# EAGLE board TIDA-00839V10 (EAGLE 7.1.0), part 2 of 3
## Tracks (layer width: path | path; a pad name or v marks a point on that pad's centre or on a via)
+5..12V
  Top 0.406: U7.3 31.36,165.84 29.82,165.84 C70.1 | U7.1 30.01,167.79 29.74,167.52 29.74,165.92 C70.1 | C70.1 29.67,165.8 D51.1 28.23,165.76 D50.1 28.26,163.91 C69.1
ACT
  Top 0.254: MSP430F67791A.29 127.51,107.38 129.01,108.88 129.01,115.62 127.26,117.38 123.01,117.38 121.51,118.88 121.51,140.62 111.01,151.12 111.01,162.62 102.76,170.88 78.43,170.88 LED_ACT.K
  Top 0.61: U8.2 110.45,181.33 108.48,183.29 96.98,183.29 93.32,179.64 74.61,179.64 JP12.1
  Bottom 0.254: 76.36,168.72 LED_ACT.K 76.32,168.77 76.32,172.5 73.09,175.73 70.96,175.73 JP12.1
AUXVCC1  (via drill 0.2, 0.4, 0.5)
  Top 0.254: v121.26,89.03 120.01,90.28 MSP430F67791A.124 120.01,98.84 108.91,109.94 v108.89,109.94 | v128.51,87.62 C26.1 | C27.1 130.66,85.22 v131.51,84.38
  Top 0.406: C26.1 128.51,84.88 128.86,85.22 C27.1
  Top 0.61: R4.2 87.17,117.8 C58.1 89.85,117.8 v89.86,117.81
  Top 0.813: R62.2 139.8,81.03 SV1.6
  Bottom 0.254: v128.51,87.62 122.66,87.62 v121.26,89.03 | v89.86,117.81 106.96,117.81 108.86,115.91 108.86,109.97 v108.89,109.94
  Bottom 0.61: v131.51,84.38 131.47,84.34 137.36,84.34 SV1.6
AUXVCC2  (via drill 0.2)
  Top 0.254: MSP430F67791A.123 119.51,89.88 v120.26,89.12 | C24.1 v125.51,86.62
  Top 0.406: C24.1 125.51,85.38 125.66,85.22 C25.1
  Bottom 0.254: v125.51,86.62 122.76,86.62 v120.26,89.12
  Bottom 0.61: v125.51,86.62 137.61,86.62 SV1.4
AUXVCC3  (via drill 0.3, 0.36, 0.4)
  Top 0.254: C43.1 128.13,97 | MSP430F67791A.3 124.76,94.38 127.41,97.03 C43.1 | C43.1 128.01,96.88 128.16,97.03 C44.1 130.16,97.03 v131.51,98.38 | v142.76,93.12 142.76,89.62 145.31,87.07 SV1.2 | R49.1 131.36,136.31 132.05,135.62 133.45,135.62 v138.66,130.41
  Top 0.406: R52.1 132.02,157.88 132.81,157.08 132.81,138.83 R49.1
  Bottom 0.254: v131.51,98.38 138.81,98.38 142.71,94.47 142.71,93.17 v142.76,93.12 142.81,93.07 144.5,93.07 145.31,93.89 145.31,128.46 143.36,130.41 v138.66,130.41
AVCC  (via drill 0.6)
  Top 0.254: 117.76,85.62 117.86,85.53 C29.1 | 118.01,86.88 117.96,86.83 C31.1 | MSP430F67791A.121 118.51,90.2 118.01,89.7 118.01,86.83 C31.1 | C31.1 117.81,86.83 117.76,86.88 117.91,87.03
  Top 0.406: C29.1 118.01,85.62 117.91,85.72 | 122.51,68.88 122.5,68.88
  Top 0.61: 122.5,68.88 116.51,74.88 116.51,78.88 117.86,80.22 | 122.51,68.88 139.26,68.88 143.26,64.88 v143.26,43.38 | 117.91,85.72 C31.1 | 117.86,80.22 117.86,85.53 | R36.2 119.2,78.89 117.86,80.22 | D36.C 127.83,43.45 v127.76,43.38 127.68,43.45 D34.C | 112.93,43.33 D32.C | v112.88,43.38 110.71,43.38 D30.C | 98.08,43.45 D28.C | 97.93,43.45 D42.C | v83.01,43.38 85.43,43.38 D40.C
  Top 0.813: D30.C 110.51,43.38 | v143.26,43.38 140.18,43.38 D38.C | 98.08,43.45 v98.01,43.38 97.93,43.45 | v112.88,43.38 112.93,43.33
  Bottom 0.61: v143.26,43.38 v127.76,43.38 v112.88,43.38 v98.01,43.38 v83.01,43.38
BTN1  (via drill 0.2, 0.4)
  Top 0.254: v121.51,98.38 MSP430F67791A.11 | R53.2 139.62,158.13 | R53.2 139.36,162.58 DBTN1.2 | R53.2 139.36,155.03 v139.51,154.88
  Bottom 0.254: v121.51,98.38 121.51,102.38 123.51,104.38 134.01,104.38 136.51,106.88 136.51,131.88 138.01,133.38 138.01,153.38 v139.51,154.88
BTN2  (via drill 0.2, 0.36)
  Top 0.254: MSP430F67791A.10 122.01,97.88 v121.51,97.38 | DBTN2.2 139.36,141.88 R50.2 139.36,136.22 v137.01,133.88
  Bottom 0.254: v121.51,97.38 121.01,97.38 120.51,97.88 120.51,102.62 123.26,105.38 133.51,105.38 135.51,107.38 135.51,132.38 v137.01,133.88
BTN3  (via drill 0.2, 0.36)
  Top 0.254: MSP430F67791A.4 123.01,94.88 v121.51,93.38 | ABTN3.2 129.66,141.78 R49.2 129.66,136.22 v132.01,133.88
  Bottom 0.254: v121.51,93.38 120.76,93.38 119.51,94.62 119.51,96.38 118.51,97.38 118.51,103.12 122.76,107.38 132.51,107.38 133.51,108.38 133.51,132.38 v132.01,133.88
BTN4  (via drill 0.2, 0.4)
  Top 0.254: MSP430F67791A.5 122.51,95.38 v121.51,94.38 | R52.2 130.01,158.23 | R52.2 129.66,162.49 ABTN4.2 | R52.2 129.66,156.22 v131.01,154.88
  Bottom 0.254: v121.51,94.38 121.01,94.38 120.51,94.88 120.51,96.62 119.51,97.62 119.51,102.88 123.01,106.38 133.01,106.38 134.51,107.88 134.51,132.88 133.01,134.38 133.01,152.88 v131.01,154.88
COM0  (via drill 0.2)
  Top 0.254: MSP430F67791A.22 121.01,103.88 v113.51,111.38 | LCD1.COM0 94.38,162.5 v109.26,147.62
  Bottom 0.254: v113.51,111.38 113.51,143.38 v109.26,147.62
COM1  (via drill 0.2)
  Top 0.254: MSP430F67791A.23 121.51,104.38 v114.51,111.38 | v109.26,149.12 109.26,149.15 96.62,161.78 96.62,162.46 LCD1.COM1
  Bottom 0.254: v114.51,111.38 114.51,143.88 v109.26,149.12
COM2  (via drill 0.2)
  Top 0.254: MSP430F67791A.24 122.01,104.88 v115.51,111.38 | LCD1.COM2 99.2,160.68 v109.26,150.62
  Bottom 0.254: v115.51,111.38 115.51,144.38 v109.26,150.62
COM3  (via drill 0.2)
  Top 0.254: MSP430F67791A.25 122.51,105.38 v116.51,111.38 | v109.26,152.12 109.26,152.19 101.7,159.75 101.7,162.46 LCD1.COM3
  Bottom 0.254: v116.51,111.38 116.51,144.88 v109.26,152.12
CUR1+
  Top 0.406: 104.04,53.12 TVS2.C 104.03,54.12 103.95,54.2 | D11.C 104.04,50.95
  Top 0.61: 103.95,54.2 103.96,54.2 R/L9.2
  Top 0.679: D3.A D11.C | 104.04,50.95 104.04,53.12
  Top 0.813: D3.A 103.96,33.36 I1+.TP
CUR1-
  Top 0.406: 107.14,53.12 TVS2.A 107.15,54.12 107.07,54.2 | D12.C 107.14,50.95
  Top 0.61: 107.07,54.2 107.06,54.2 R/L10.2
  Top 0.679: D4.A D12.C | 107.14,50.95 107.14,53.12
  Top 0.813: D4.A 107.06,33.41 I1-.TP
CUR2+
  Top 0.406: TVS3.C 118.73,53.99 | 118.73,53.99 118.86,54.12 | 118.73,53.99 118.86,54.12
  Top 0.61: 118.86,54.12 118.83,54.12 R/L11.2 | D13.C 118.83,53.12 TVS3.C
  Top 0.679: D5.A D13.C
  Top 0.813: D5.A 118.83,33.41 I2+.TP
CUR2-
  Top 0.406: TVS3.A 121.98,54.12 | TVS3.A 121.97,53.12 121.93,53.09 | TVS3.A 121.94,54.12
  Top 0.61: 121.98,54.12 121.93,54.12 R/L12.2
  Top 0.679: D6.A D14.C 121.93,53.09
  Top 0.813: D6.A 121.93,33.36 I2-.TP
CUR3+
  Top 0.406: 133.7,54.12 TVS4.C 133.71,53.12
  Top 0.61: 133.7,54.12 133.71,54.12 R/L13.2
  Top 0.679: 133.71,53.12 D15.C D7.A
  Top 0.813: D7.A 133.71,33.47 I3+.TP
CUR3-
  Top 0.406: 136.82,54.12 TVS4.A 136.81,53.12
  Top 0.61: 136.82,54.12 136.81,54.12 R/L14.2
  Top 0.679: 136.81,53.12 D16.C D8.A
  Top 0.813: D8.A 136.81,33.3 I3-.TP
CURN+
  Top 0.406: 88.94,53.12 TVS1.C 88.86,54.02 | 88.86,54.02 88.95,54.12 | 88.96,53.92 88.86,54.02
  Top 0.61: 88.95,54.12 88.96,54.12 R/L7.2
  Top 0.679: D1.A D9.C 88.96,53.92
  Top 0.813: D1.A 88.96,33.31 IN+.TP
CURN-
  Top 0.406: 92.16,53.24 92.04,53.12 | 92.16,53.24 TVS1.A 92.07,54.12 | 92.06,53.14 92.16,53.24
  Top 0.61: 92.07,54.12 92.06,54.12 R/L8.2
  Top 0.679: D2.A D10.C 92.06,53.14
  Top 0.813: D2.A 92.06,33.45 IN-.TP
DRESET  (via drill 0.36)
  Top 0.254: v49.01,120.88 49.51,120.38 89.51,120.38 91.01,118.88 91.01,102.88 v91.13,102.75 | MSP430F67791A.102 106.51,93.38 v104.63,91.5
  Bottom 0.254: JP5.2 27.99,127.81 42.08,127.81 v49.01,120.88 | v91.13,102.75 91.13,96.75 96.38,91.5 v104.63,91.5
DRV1GND
  Top 0.254: MSP430F67791A.20 148.39,102.88 152.73,98.53
  Top 0.61: U1GND.1 36.38,2.54 37.11,1.81 124.41,1.81 152.73,30.13 152.73,98.53
DRV2GND
  Top 0.254: MSP430F67791A.18 146.49,101.88 150.75,97.62
  Top 0.61: U2GND.1 63.15,5.24 64.89,3.49 123.11,3.49 150.75,31.12 150.75,97.62
DRV3GND
  Top 0.254: MSP430F67791A.12 126.3,98.88 127.33,99.91 143.23,99.91 147.62,95.51
  Top 0.61: U3GND.1 100.68,7.05 100.96,6.77 121.46,6.77 147.57,32.88 147.57,95.46 147.62,95.51
DRV4GND
  Top 0.254: MSP430F67791A.95 95.09,96.88 90.63,92.41 90.63,75.78 90.09,75.24 67.21,75.24 66.57,75.88 66.57,76.97 65.7,77.84 U4GND.1
DRV5GND
  Top 0.254: MSP430F67791A.93 94.16,97.88 89.46,93.18 89.46,78.32 88.39,77.25 U5GND.1
DRV6GND
  Top 0.254: U6GND.1 66.47,87.84 67,88.38 74.01,88.38 75.39,88.38 78.36,85.4 80.13,85.4 85.77,85.4 85.93,85.56 86.46,86.09 87.35,86.98 87.35,94.22 93.51,100.38 MSP430F67791A.88
DRV123OUTA  (via drill 0.36)
  Top 0.254: 149.25,96.81 145.26,100.8 126.11,100.8 125.19,99.88 MSP430F67791A.14
  Top 0.305: 149.25,96.81 149.25,32.16 122.22,5.14 95.15,5.14 v93.24,7.04
  Top 0.61: U1OUT.1 30.16,6.17 v30.12,6.13 | v54.73,6.18 56.27,6.18 U2OUT.1 | U3OUT.1 93.76,7.56 v93.24,7.04
  Bottom 0.61: v30.12,6.13 54.68,6.13 v54.73,6.18 56.27,6.18 57.13,7.04 v93.24,7.04
DRV123OUTB
  Top 0.254: 149.96,97.24 145.97,101.23 125.58,101.23 124.72,100.38 MSP430F67791A.15
  Top 0.305: U$7.3 76.17,5.35 77.16,4.35 122.5,4.35 149.96,31.81 149.96,97.24
DRV456OUTA  (via drill 0.5)
  Top 0.254: U6OUT.1 71.69,86.18 73.89,83.98 77.59,83.98 | MSP430F67791A.89 93.74,99.88 88.4,94.53 87.98,94.11 87.93,94.06 87.93,84.49 87.42,83.98 v78.1,83.98
  Top 0.305: U4OUT.1 59.67,74.44 v59.97,74.15 | v79.14,80.86 76.21,80.86 U5OUT.1 77.64,80.88 v78.28,81.52 | v78.1,83.98 77.59,83.98
  Bottom 0.305: v59.97,74.15 79.04,74.15 80.11,75.22 80.11,79.89 v79.14,80.86 | v78.28,81.52 78.28,83.8 v78.1,83.98
DRV456OUTB
  Top 0.254: MSP430F67791A.94 94.62,97.38 89.99,92.74 89.99,76.13 89.56,75.7 69.59,75.7 69.19,76.11 U$8.3
DRVOUT1  (via drill 0.36)
  Top 0.254: MSP430F67791A.21 149.26,103.38 153.54,99.09
  Top 0.305: U$7.1 v67.75,8.43 v67.74,8.44 | v35.28,7.58 U1OUT.3 | U1OUT.3 | U1OUT.3 33.56,3.18 35.63,1.1 125.12,1.1 153.54,29.52 153.54,99.09
  Bottom 0.305: v67.74,8.44 36.14,8.44 v35.28,7.58
DRVOUT2  (via drill 0.36)
  Top 0.254: MSP430F67791A.19 147.41,102.38 151.71,98.08 | U$7.2 75.67,7.48 v73.45,5.27 | v61.97,5.75 61.97,6.79 61.64,7.12 60.61,7.12 U2OUT.3
  Top 0.305: U2OUT.3 60.66,6.71 60.66,3.73 61.75,2.65 123.72,2.65 151.71,30.64 151.71,98.08
  Bottom 0.254: v73.45,5.27 62.46,5.27 v61.97,5.75
DRVOUT3  (via drill 0.36)
  Top 0.254: U$7.5 76.67,11.53 v76.96,11.82 | v97.18,11.49 97.18,10.11 U3OUT.3 | MSP430F67791A.13 125.93,99.38 126.9,100.34 144.4,100.34 148.49,96.25
  Top 0.305: U3OUT.3 97.16,6.33 97.58,5.9 121.89,5.9 148.49,32.5 148.49,96.25
  Bottom 0.254: v76.96,11.82 96.85,11.82 v97.18,11.49
DRVOUT4  (via drill 0.5)
  Top 0.254: U$8.1 | 63.53,76.24 64.07,76.24 64.56,75.75 65.12,75.19 65.15,75.19 65.56,74.79 90.55,74.79 91.16,75.4 91.16,91.96 95.58,96.38 MSP430F67791A.96
  Top 0.305: 63.53,76.24 U4OUT.3 | U$8.1 68.17,76.36 v68.02,76.21 | v65.48,76.21 65.02,76.21 64.56,75.75
  Bottom 0.305: v68.02,76.21 v65.48,76.21
DRVOUT5
  Top 0.254: U5OUT.3 72.79,81.95 73.4,82.56 88.06,82.56 88.11,82.61 88.48,82.98 88.95,83.45 88.95,93.56 94.27,98.88 MSP430F67791A.91
  Top 0.305: U$8.2 68.68,77.66 68.96,77.94 71.55,77.94 72.74,79.13 72.74,80.83 U5OUT.3
DRVOUT6
  Top 0.254: U6OUT.3 71.87,82.78 71.87,82.81 72.29,83.22 87.83,83.22 88.11,83.5 88.36,83.75 88.47,83.85 88.47,93.91 93.93,99.38 MSP430F67791A.90
  Top 0.305: U$8.5 69.68,82.02 U6OUT.3
DRVPOWER1  (via drill 0.36)
  Top 0.61: R40.1 31.23,13.46 U$1.1 31.48,13.71 C41.1 | R41.1 58.63,12.84 U$2.1 58.65,13.64 v57.86,14.44 58.31,14.89 C42.1 | R44.1 95.28,16.3 U$3.1 95.45,17.73 95.6,17.89
  Top 0.813: v94.84,17.89 95.6,17.89 96.47,17.89 C51.1 | R67.2 v82.75,12.81 | 57.92,14.38 v57.86,14.44 | C41.1 30.25,15.4 v30.22,15.43
  Bottom 0.813: DRV-I.1 147.99,72.75 153.64,67.09 153.64,28.71 142.82,17.89 v94.84,17.89 88.59,17.89 83.51,12.81 v82.75,12.81 81.13,14.44 v57.86,14.44 56.87,15.43 v30.22,15.43
DRVPOWER4  (via drill 0.5)
  Top 0.254: v60.93,83.45 64.11,83.45 66.25,81.3 R68.2
  Top 0.61: 59.25,80.58 R45.1 | R45.1 59.11,80.8 | v60.93,83.45 60.45,82.96 C52.1 59.5,82.14 59.1,81.75 R45.1 | U$4.1 59.24,80.3 R45.1
  Bottom 0.61: 68.33,86.66 U$6.1 | C55.1 67.69,87.3 U$6.1 | U$6.1 68.45,86.54 R64.1 74.88,86.54 76.71,84.72 | 76.71,84.72 76.71,81 R47.1 77.06,80.42 77.01,80.38 U$5.1 77.42,78.81 C54.1 | 76.71,84.72 78.71,86.72 85.14,86.72 87.32,88.91 DRV-I1.1
  Bottom 0.813: v60.93,83.45 64.11,83.45 64.89,84.23 64.89,86.8 65.28,87.18 66.36,87.18 C55.1
DTCK  (via drill 0.36)
  Top 0.254: v50.01,121.38 50.51,120.88 89.76,120.88 91.51,119.12 91.51,103.88 v91.88,103.5 | MSP430F67791A.101 105.51,93.88 v103.88,92.25
  Bottom 0.254: JP6.2 27.99,130.35 34.88,130.35 36.67,128.56 42.83,128.56 v50.01,121.38 | v103.88,92.25 96.68,92.25 91.72,97.21 91.72,103.33 v91.88,103.5
DTDI  (via drill 0.36)
  Top 0.254: v52.01,122.38 52.51,121.88 90.26,121.88 92.51,119.62 92.51,105.88 v93.38,105 | MSP430F67791A.99 103.51,94.88 v102.38,93.75
  Bottom 0.254: JP8.2 28.08,135.34 32.84,135.34 35.13,133.05 41.33,133.05 v52.01,122.38 | v93.38,105 93.38,98.34 98.02,93.71 102.34,93.71 v102.38,93.75
DTDO  (via drill 0.36)
  Top 0.254: v53.01,122.88 53.51,122.38 90.51,122.38 93.01,119.88 93.01,106.57 v93.93,105.65 | MSP430F67791A.98 102.51,95.38 v101.63,94.5
  Bottom 0.254: JP9.2 27.99,137.97 31.74,137.97 35.64,134.07 39.67,134.07 | 39.67,134.07 39.7,134.07 | 39.67,134.07 39.69,134.06 41.83,134.06 v53.01,122.88 | v101.63,94.5 101.55,94.42 98.5,94.42 94.13,98.79 94.13,105.44 v93.93,105.65
DTMS  (via drill 0.36)
  Top 0.254: v51.01,121.88 51.51,121.38 90.01,121.38 92.01,119.38 92.01,104.88 v92.63,104.25 | MSP430F67791A.100 104.51,94.38 v103.13,93
  Bottom 0.254: JP7.2 27.99,132.89 33.84,132.89 37.17,129.56 43.33,129.56 v51.01,121.88 | v92.63,104.25 92.63,97.49 97.23,92.9 103.03,92.9 v103.13,93
DVCC  (via drill 0.36, 0.5, 0.6)
  Top 0.254: MSP430F67791A.126 121.01,90.78 121.91,89.88 C35.1
  Top 0.305: R51.1 33.67,138.06 26.09,145.59 JP10.2
  Top 0.406: 123.51,88.38 C33.1 124.01,88.28 | R53.1 137.66,166.53 140.01,168.88 | R50.1 137.66,146.38 141.98,150.71 | U5.1 43.74,181.25 C78.2 46.32,179.37 v48.46,177.22
  Top 0.61: 124.01,88.28 v124.01,78.88 121.88,78.88 | C33.1 C35.1 | 58.4,164.38 v58.5,164.28 R54.1 | U8.1 v113.76,182.6 112.03,182.6 C79.1 | v110.34,176.64 v113.89,176.64 | R55.1 v63.95,164.28 | R56.1 v69.03,164.28 | R57.1 v74.11,164.28 | R58.1 v86.81,164.28 | R59.1 v91.89,164.28 | R60.1 v96.97,164.28 | R61.1 v102.31,164.28
  Top 0.813: JP3.2 80.09,105.38 81.09,106.38 v81.09,118.43 | DVCC.1 DVCC.2 DVCC.3 DVCC.4 | 121.88,78.88 R36.1 | 124.05,78.92 v124.01,78.88 131.11,78.88 136.93,84.69 136.93,88.8 142.01,93.88 142.01,97.09 v141.98,97.11 | v81.09,118.43 | v103.33,179.79 114.24,168.88 140.01,168.88 141.98,166.9 141.98,150.71 v141.98,109.18
  Bottom 0.406: v48.46,177.22 51.84,177.22 52.37,176.69
  Bottom 0.61: v102.31,164.28 v96.97,164.28 v91.89,164.28 v86.81,164.28 v74.11,164.28 v69.03,164.28 v63.95,164.28 v58.5,164.28 | R66.2 87.27,105.95 86.54,106.69 81.2,106.69 80.16,105.64 80.16,104.03 | v103.33,179.79 107.19,179.79 v110.34,176.64 | 113.76,177.53 113.89,177.4 v113.89,176.64 113.76,176.77 v113.76,182.6
  Bottom 0.813: 47.01,145.05 47.01,162.69 48.61,164.3 48.63,164.28 50.43,164.28 | v81.09,118.43 81.09,119.97 77.69,123.38 56.51,123.38 47.01,132.88 47.01,145.05 | JP10.2 24.18,145.57 24.17,145.56 | 80.16,104.03 JP3.2 | R63.2 129.11,78.57 128.8,78.88 v124.01,78.88 | v141.98,97.11 v141.98,109.18 | 24.33,145.73 46.05,145.73 46.19,145.87 | v103.33,179.79 62.94,179.79 | 62.94,179.79 55.47,179.79 52.37,176.69 51.61,175.93 51.61,165.28 | v58.5,164.28 50.43,164.28 | 46.19,145.87 46.91,146.59 | 46.96,144.87 46.18,145.65 46.33,145.65 46.37,145.69 | 47.01,145.05 46.37,145.69 | 46.37,145.69 46.19,145.87 | DVCC.1 63.13,179.98 62.94,179.79 | 51.18,164.85 52.02,164.85 | 51.61,165.54 51.61,165.46 50.71,164.56 | 50.43,164.28 50.42,164.27 | 51.59,165.57 51.74,165.41 | 51.74,165.41 52.78,164.37 | 50.43,164.28 50.71,164.56 | 50.71,164.56 50.89,164.56 51.18,164.85 | 51.61,165.28 51.74,165.41 | 51.61,165.28 51.18,164.85 | 51.13,164.85 51.18,164.85
  Bottom 1.27: 24.33,145.73 JP10.2
DVSYS_VDSYS  (via drill 0.2, 0.4, 0.5)
  Top 0.254: 129.26,89.9 C34.1 128.23,88.88 v126.76,88.88 | C36.1 106.28,113.75 106.81,113.75 108.05,112.5 108.41,112.5 109.27,111.64 109.27,110.62 110.01,109.89 110.01,109.88 120.51,99.44 MSP430F67791A.125 120.51,90.53 122.36,88.88 v122.51,88.88 | MSP430F67791A.69 106.51,109.88 v106.26,109.62
  Top 0.406: 129.26,89.9 130.48,89.9 v131.76,88.62
  Top 0.61: DRVPWR4.1 v89.02,111.46 | v106.26,112.62 C36.1
  Top 0.813: DRVPWR1.1 141.41,75.03 SV1.1
  Bottom 0.254: v122.51,88.88 v126.76,88.88
  Bottom 0.61: v131.76,88.62 146.23,88.62 147.04,87.82 147.04,80.65 SV1.1 | v89.02,111.46 105.67,111.46 106.26,110.88 | 106.26,110.88 v106.26,109.62 | 106.26,110.88 v106.26,112.62
EXT
  Top 0.813: JP10.3
  Top 1.016: JTAG.4 19.39,141.78 20.67,143.06 JP10.3
GND  (via drill 0.3, 0.36, 0.4, 0.41, 0.5, 0.6)
  Top 0.254: MSP430F67791A.70 108.77,109.38 108.94,109.2 108.94,106.69 v109.51,106.12
  Top 0.61: R65.1 54.84,76.49 56.74,74.58
  Top 0.813: R39.1 75.29,97.47 75.29,97.52 77.83,97.52 | 77.83,97.52 77.83,97.61 | 78.4,100.38 78.33,100.31 78.33,98.03 77.83,97.52 | 77.83,97.52 77.8,97.54
  Top 1.016: C9.2 52.11,62.27 R32.2 R15.2 | R17.2 R33.2 66.91,62.17 C11.2 | R19.2 R34.2 79.16,62.17 C13.2 | L6.2 82.57,46.38 82.65,46.47
  Bottom 1.016: C67.2 82.88,90.76 C68.2
  Bottom 1.27: 80.8,90.82 C67.2
  other vias: 105.32,109.67 128.01,112.38 129.51,119.38 109.95,100.24 130.51,121.38 132.51,124.88 125.76,97.62 130.76,93.62 134.51,95.62 134.51,91.62 109.51,105.12 107.01,118.88 107.01,122.88 86.51,148.38 74.01,148.38 61.51,148.38 88.99,119.17 124.65,75.28 125.26,72.23 86.51,141.38 74.01,141.38 61.51,141.38 130.26,88.67 132.51,127.38 132.51,129.38 132.51,131.38 112.26,93.12 116.26,93.12 120.26,82.88 110.51,81.38 121.76,82.88 121.76,81.38 120.26,81.38 120.38,64.88 135.26,64.88 98.01,63.88 98.01,59.38 98.01,54.38 112.95,63.89 112.95,59.39 112.95,54.39 127.82,63.89 127.82,59.39 127.82,54.39 90.51,60.12 90.51,58.38 90.51,64.88 105.51,64.88 105.51,60.12 105.51,58.38 120.38,60.12 120.38,58.38 135.26,60.12 135.26,58.38 141.26,54.38 81.96,60.22 120.26,75.38 121.76,75.38 101.19,86.44 96.44,81.69 96.44,86.44 110.26,93.12 96.43,89.44 101.19,89.44 101.19,81.69 114.76,93.12 69.77,58.69 57.58,58.44 47.84,60.94 81.13,65.01 74.78,60.94 119.06,88.08 117.66,95.03 114.36,94.72 112.26,94.62 66.06,78.5 70.56,76.67 71.9,76.77 74.76,90.27 75.75,90.27 75.78,89.44 74.81,89.41 79.16,88.95 81.8,89.1 83.73,89.46 73.54,89.1 82.81,89.31 80.4,89.18 100.29,54.38 95.47,54.38 98.01,61.66 112.99,61.66 127.73,61.66 145.51,61.66 145.51,64.45 145.6,58.88 110.41,54.39 115.74,54.39 125.54,54.39 130.36,54.39 98.01,50.31 98.01,46.76 112.99,50.56 113.25,46.5 90.39,46.76 90.39,41.42 98.26,41.42 105.63,46.76 105.63,41.67 120.36,46.5 120.36,41.67 135.09,46.5 135.09,41.93 96.44,83.97 101.19,83.97 96.44,79.14 101.19,79.14 44.61,175.03 44.61,173.25 44.61,170.97 46.64,170.97 46.64,173.25 46.64,175.03 145.6,56.34 145.6,53.29 145.6,50.24 145.6,47.2 113.76,12.46 118.58,12.46 113.76,9.42 118.58,9.42 82.51,10.18 86.83,10.18 82.51,5.61 86.83,5.61 53.52,68.34 109.95,102.52 109.95,104.05 111.48,104.05 113.51,107.86 118.84,111.41 120.62,111.41 114.27,96.43 114.27,98.46 114.27,100.49 117.57,99.98 117.57,98.46 117.57,96.43 112.26,96.4 110.23,94.62 110.23,96.4 43.4,12.21 47.72,12.21 43.4,4.08 47.72,4.08 66.26,11.45 70.58,11.45 113.76,15 118.58,15 138.65,10.43 143.47,10.43 138.65,7.89 143.47,7.89 138.65,4.84 143.47,4.84 62.81,78.42 63.52,82.53 67.61,82.94
  pour Bottom (rank 2): 147.8,0.49 29.44,0.49 25.5,4.43 25.5,13.45 28.42,16.37 80.11,16.37 82.4,18.65 82.4,56.24 81.76,56.88 46.71,56.88 46.45,57.13 46.45,65.64 55.6,74.79 56.36,74.79 58.27,76.69 58.27,82.03 60.17,83.93 63.22,83.93 63.98,84.69 63.98,86.6 65.89,88.5 71.73,88.5 75.54,92.31 75.54,118.86 75.28,119.11 46.96,119.11 43.53,122.54 12.42,122.54 11.66,123.3 11.66,137.52 12.16,138.03 21.69,138.03 22.2,138.54 22.2,149.59 22.96,150.35 43.15,150.35 43.15,185.78 45.82,185.91 114.91,185.91 115.16,185.66 115.16,171.69 117.32,169.53 152.12,169.53 155.55,166.1 155.55,16.62 154.15,15.22 149.45,15.22 147.8,13.57
  pour Top (rank 2): 147.8,0.49 29.44,0.49 25.5,4.43 25.5,13.45 28.42,16.37 80.11,16.37 82.4,18.65 82.4,56.24 81.76,56.88 46.71,56.88 46.45,57.13 46.45,65.64 55.6,74.79 56.36,74.79 58.27,76.69 58.27,82.03 60.17,83.93 63.09,83.93 63.98,84.82 63.98,86.6 65.89,88.5 71.73,88.5 75.54,92.31 75.54,118.86 75.28,119.11 46.84,119.11 43.41,122.54 12.42,122.54 11.66,123.3 11.66,137.52 12.16,138.03 21.69,138.03 22.2,138.54 22.2,149.59 22.96,150.35 43.15,150.35 43.15,185.53 45.95,185.91 114.91,185.91 115.16,185.66 115.16,171.69 117.32,169.53 152.25,169.53 155.55,166.23 155.55,16.62 154.15,15.22 149.45,15.22 147.8,13.57
  pour Bottom (no thermals): 85.6,91.85 79.53,91.85 78.61,90.92 78.15,90.92 77.95,91.12 76.91,91.12 76.45,90.66 68.63,90.66 67.23,89.26 63.57,89.26 63.12,88.81 61.64,88.81 61.31,88.48 61.31,85.61 62.13,84.79 62.89,84.79 63.29,85.2 63.29,86.77 64.97,88.45 83.56,88.45 85.8,90.69 85.8,91.78
GND_RS232  (via drill 0.36)
  other vias: 24.86,180.45 24.86,179.43 24.86,178.42 24.86,177.4 24.86,176.39 24.86,173.59 24.86,170.04 24.86,169.02 24.86,168 24.86,166.99 26.13,169.02 26.13,168 26.13,166.99 27.4,168 27.4,166.99 25.37,161.4 25.37,159.37 25.37,156.83 27.4,156.83 29.69,156.83 29.69,155.56 27.66,155.56 25.37,155.81 32.99,161.15 31.04,157.21 37.79,157.18 37.31,155.3 37.31,161.15 32.99,162.67 37.31,162.92 34.26,162.67 34.26,161.15 37.31,164.45 37.31,165.97 37.31,167.5 38.07,169.02 37.06,172.32 26.9,180.45 28.93,180.45 28.93,181.97 35.53,171.81 28.93,184.01 31.47,184.26 31.47,182.48 22.07,184.51 13.69,184.26 13.18,154.8 17.75,154.8 21.82,154.8
  pour Top: 11.4,154.29 11.4,186.8 38.83,186.8 38.83,154.29
  pour Bottom: 11.4,155.56 11.4,186.8 38.83,186.8 38.83,154.29 11.4,154.29
I1+
  Top 0.254: MSP430F67791A.114 115.01,89.38 114.51,88.88 114.51,83.38 113.51,82.38
  Top 0.406: 113.51,82.38 110.51,79.38 110.51,70.88 107.06,67.42 C17.1
  Top 0.61: C16.1 103.86,63.88 R26.2
  Top 0.679: C16.1 C17.1
I1-
  Top 0.254: MSP430F67791A.115 115.51,89.12 115.01,88.62 115.01,82.88 114.01,81.88
  Top 0.406: 114.01,81.88 111.51,79.38 111.51,70.38 108.96,67.83 C17.2
  Top 0.61: C5.1 108.96,61.62 | 108.96,61.62 R27.2 | 108.96,61.62 C17.2
I2+
  Top 0.254: C18.1 119.07,64.47 | MSP430F67791A.116 116.01,88.88 115.51,88.38 115.51,82.38 114.51,81.38
  Top 0.4: 118.88,65.38 118.88,66.5 112.51,72.88
  Top 0.406: 114.51,81.38 112.51,79.38 112.51,72.88 | 118.88,65.38 118.88,63.92 C18.1
  Top 0.61: C18.1 118.73,63.88 R28.2
  Top 0.679: C18.1 C19.1
I2-
  Top 0.254: MSP430F67791A.117 116.51,88.62 116.01,88.12 116.01,81.88 115.01,80.88
  Top 0.406: 115.01,80.88 113.51,79.38 113.51,73.38 121.01,65.88 123.38,65.88 123.83,65.42 C19.2
  Top 0.61: C19.2 123.73,63.88 R29.2 123.73,59.38 C6.1
I3+
  Top 0.254: MSP430F67791A.118 117.01,88.38 116.51,87.88 116.51,81.38 115.51,80.38
  Top 0.406: 115.51,80.38 114.51,79.38 114.51,73.88 121.51,66.88 132.26,66.88 133.71,65.42 C20.1
  Top 0.61: C20.1 133.61,63.88 R30.2
  Top 0.679: C20.1 C21.1
I3-
  Top 0.254: MSP430F67791A.119 117.51,88.12 117.01,87.62 117.01,80.88 116.01,79.88
  Top 0.406: 116.01,79.88 115.51,79.38 115.51,74.38 122.01,67.88 136.26,67.88 138.71,65.42 C21.2
  Top 0.61: C21.2 138.61,63.88 R31.2 138.61,59.38 C7.1
IN+
  Top 0.254: MSP430F67791A.109 112.51,89.38 108.51,85.38 108.51,83.88
  Top 0.305: C15.1 92.38,64.27
  Top 0.406: 108.51,83.88 108.51,71.88 103.51,66.88 93.51,66.88 92.01,65.38 92.01,63.88 C15.1
  Top 0.61: C14.1 88.86,63.88 R24.2
  Top 0.679: C14.1 92.01,63.88
IN-
  Top 0.254: MSP430F67791A.110 113.01,89.12 109.51,85.62 109.51,83.88
  Top 0.305: C15.2 94.29,64.27
  Top 0.406: 109.51,83.88 109.51,71.38 104.01,65.88 94.51,65.88 93.96,65.33 C15.2
  Top 0.61: C15.2 93.86,63.88 R25.2 93.96,61.62 C4.1
INT
  Top 1.016: JTAG.2 18.43,144.32 22.24,148.13 JP10.1
LED1
  Top 0.254: MSP430F67791A.28 127.76,106.88 129.51,108.62 129.51,115.88 127.51,117.88 123.26,117.88 122.01,119.12 122.01,140.88 111.51,151.38 111.51,162.88 103.01,171.38 73.85,171.38 LED1.K
LED2
  Top 0.254: MSP430F67791A.27 128.01,106.38 130.01,108.38 130.01,116.12 127.76,118.38 123.51,118.38 122.51,119.38 122.51,141.12 112.01,151.62 112.01,163.12 103.26,171.88 69.27,171.88 LED2.K
LED3
  Top 0.254: MSP430F67791A.26 128.26,105.88 130.51,108.12 130.51,116.38 128.01,118.88 123.76,118.88 123.01,119.62 123.01,141.38 112.51,151.88 112.51,163.38 103.51,172.38 64.69,172.38 LED3.K
LED4
  Top 0.254: MSP430F67791A.45 119.01,136.88 110.01,145.88 110.01,162.12 102.26,169.88 90.01,169.88 88.98,168.84 LED4.K
LED5  (via drill 0.36)
  Top 0.254: MSP430F67791A.43 120.01,138.67 v118.79,139.89
  Bottom 0.254: v118.79,139.89 118.79,145.65 112.62,151.82 112.62,163.79 106.35,170.06 95.39,170.06 LED5.K
LED6  (via drill 0.36)
  Top 0.254: MSP430F67791A.44 119.51,137.47 v117.65,139.33
  Bottom 0.254: v117.65,139.33 117.65,146.03 111.86,151.82 111.86,163.33 106.32,168.87 99.28,168.87 LED6.K
LINE1
  Top 1.016: 16.36,39.53 L1.1 16.28,39.53 | 16.28,39.53 16.36,39.61 | 16.28,39.53 16.21,39.46 16.21,36.71 16.36,36.56 16.27,36.47 R1.2 | R1.2 16.27,36.39 16.36,36.3 16.21,36.16 | LINE1.TP 16.21,36.34 R1.2
LINE2
  Top 1.016: L3.1 41.57,40.05 41.76,39.86 41.67,39.77 R2.2 41.96,36.38 LINE2.TP
LINE3
  Top 1.016: R3.2 68.09,36.64 68.17,36.56 67.71,36.1 | L5.1 68.11,39.67 68.17,39.61 68.09,39.52 R3.2 | LINE3.TP 67.71,36.28 R3.2
N$1
  Top 0.813: D24.A 137.24,79.12 R62.1
N$2  (via drill 0.36)
  Top 0.813: D25.A 125.91,77.22 v125.88,77.25
  Bottom 0.813: v125.88,77.25 127.25,77.25 R63.1
N$4
  Top 0.254: R56.2 72.05,165.34 LED1.A
N$6
  Top 0.61: R24.1 R20.2 87.16,57.23 R/L7.1
N$7
  Top 0.254: R55.2 66.97,165.34 LED2.A
N$8
  Top 0.61: R6.2 12.87,45.54 12.88,45.55 12.93,45.5 R5.1
N$9
  Top 0.813: DRVPWR1.3 130.75,75.07 D25.C 130.9,77.06 D24.C
N$10
  Top 0.254: JP4.1 27.99,127.81 22.14,127.81 21.62,128.33 R48.2
N$11
  Top 0.61: U1GND.2 36.36,12.68 U$1.3 33.38,13.04 C41.2
N$12
  Top 0.61: U2GND.2 62.77,11.91 U$2.3 61.3,12.22 C42.2
N$13
  Top 1.016: 11.05,48.98 11.02,49.01 | 11.05,48.98 R7.2 | R6.1 11.15,48.88 11.05,48.98
N$14
  Top 0.679: R14.2 R15.1
  Top 1.016: R14.2 52.01,56.21 51.16,55.35 13.56,55.35 11.02,52.81 11.02,51.04 11.05,51.01 R7.1
N$15
  Top 1.016: 37.74,46.42 37.69,46.47 | R9.2 37.74,46.42 | R8.1 37.82,46.34 37.74,46.42
N$16
  Top 1.016: R10.2 36.02,49.62 35.92,49.51 36.04,49.39 R9.1
N$17
  Top 0.254: U3.5 54.82,108.04 R38.2
N$18
  Top 1.016: R92.2 7.24,104.09 7.21,104.12 7.25,104.16 D18.A 3.11,104.34 2.9,104.12 2.75,104.27 D17.C
N$19
  Top 0.679: R16.2 R17.1
  Top 1.016: R16.2 64.01,55.25 62.08,53.32 36.68,53.32 36.17,52.81 36.17,52.05 35.92,51.8 36.02,51.7 R10.1
N$20
  Top 0.61: D3.C 100.51,36.88
  Top 0.813: 100.51,36.88 D28.A
N$21
  Top 0.254: R59.2 88.13,165.34 LED4.A
N$22
  Top 0.61: U$3.3 97.79,17.31 C51.2
  Top 0.813: U3GND.2 98.37,14.93 U$3.3
N$23
  Top 0.61: D29.C 100.51,50.83 D11.A
  Top 0.813: D11.A 100.51,50.88
N$24
  Top 0.61: 64.21,79.62 U4GND.2 64.09,79.34 U$4.3 62.81,80.18 62.23,80.75 62.23,82.02 C52.2
N$25
  Top 0.61: R30.1 R23.2 131.81,59.27 R/L13.1
N$26
  Top 0.61: U5GND.2 75.7,79.17 U$5.2
  Bottom 0.61: 75.78,79.25 U$5.2 75.52,79 C54.2
N$27
  Top 0.254: R60.2 93.21,165.34 LED5.A
N$28
  Top 0.61: U6GND.2 68.22,85.44 U$6.2
  Bottom 0.61: 68.27,85.45 U$6.2 68.18,85.4 C55.2
N$29
  Top 1.016: R12.2 64.32,45.66 64.36,45.7 64.4,45.67 R11.1
N$30
  Top 0.254: R54.2 61.89,165.34 LED3.A
N$31
  Top 0.61: R28.1 R22.2 117.03,57.12 R/L11.1
N$32
  Top 0.61: R26.1 R21.2 102.06,59.27 R/L9.1
N$33
  Top 1.016: R12.1 62.49,45.86 62.59,45.96 62.49,46.05 R13.2
N$34
  Top 0.679: R18.2 R19.1
  Top 1.016: R13.1 72.26,50.55 76.3,54.59 76.3,57.39 76.26,57.43 R18.2
N$35
  Top 0.813: DRVPWR1.2 132.4,72.98 DRV-I.2
N$36
  Top 0.254: R61.2 98.29,165.34 LED6.A
N$37
  Top 0.254: U3.4 53.5,110.37 53.01,109.88 C45.1
N$38
  Top 0.254: U3.3 53.26,110.88 52.26,109.88 51.36,109.88 R35.1 R37.2
N$39
  Top 0.813: D4.C 110.51,36.88 D30.A
N$40
  Top 0.813: D31.C 110.46,48.83 D12.A
N$41
  Top 0.61: 59.17,78.67 R45.2 59.14,78.7 59.92,78.7 60.22,78.39 U$4.2 60.48,78.38 60.48,77.71 61.37,76.81 U4OUT.2
N$42
  Top 0.813: D5.C 115.51,36.88 D32.A
N$43
  Top 0.61: U5OUT.2 74.49,79.23 U$5.3
  Bottom 0.61: U$5.3 74.47,80.47 R47.2
N$44
  Top 0.254: R58.2 83.05,165.34 LED_REACT.A
N$45
  Top 0.305: U$7.7 U$7.6
N$46
  Top 0.254: R57.2 77.13,165.34 LED_ACT.A
N$47
  Top 1.016: 23.07,103.73 D20.A 22.93,103.79 22.83,103.69 22.56,103.44 20.8,101.68 | D19.C 18.9,103.87 20.8,101.97 20.8,101.68 | R93.2 20.8,101.68
N$49
  Top 0.61: D26.A 87.06,116.21 R4.1
N$50
  Top 0.305: U$8.6 U$8.7
N$51  (via drill 0.5)
  Top 0.61: D27.A v87.22,100.59
  Bottom 0.61: v87.22,100.59 87.22,102.97 R66.1
N$52
  Top 0.61: D27.C 87.32,105.62 DRVPWR4.3 87.19,107.93 85.98,107.93 85.09,108.82 D26.C
N$53
  Top 0.61: DRVPWR4.2 87.78,109.76 87.81,109.79 88.97,109.79 89.51,109.25 89.51,100.95 DRV-I1.2
N$54
  Top 0.813: D33.C 115.43,48.83 D13.A
N$55
  Top 0.61: U6OUT.2 68.53,84.48 U$6.3
  Bottom 0.61: U$6.3 68.7,84.2 69.24,84.74 70.3,84.74 R64.2
N$56
  Top 0.254: U$7.8 75.17,12.71 C57.1 75.27,12.81 R67.1
N$58
  Top 0.305: U$8.8 68.1,79.6 R68.1 66.6,79.63 66.6,80.27 66.75,80.42 67.59,80.42 67.98,80.82 C56.1
N$62
  Top 0.813: D6.C 125.26,36.88 D34.A
N$63
  Top 0.813: D35.C 125.33,48.83 D14.A
N$64
  Top 0.813: D7.C 130.51,36.88 D36.A
N$65
  Top 0.61: U1OUT.2 31.86,11.27 U$1.2 31.37,11.76 R40.2
N$66
  Top 0.813: 130.38,50.88 D15.A 130.38,50.8 D37.C
N$67
  Top 0.61: U2OUT.2 58.73,10.88 U$2.2 58.47,11.14 R41.2
N$68
  Top 0.61: U3OUT.2 95.46,14.55 U$3.2 95.41,14.6 R44.2
N$70
  Top 0.813: D8.C 140.21,39.85 D38.A
N$73
  Top 0.813: D39.C 140.13,50.8 D16.A
N$74
  Top 0.813: D1.C 85.56,40 D40.A
N$75
  Top 0.813: D41.C 85.51,50.83 D9.A
N$76
  Top 0.813: D2.C 95.46,39.98 D42.A
N$77
  Top 0.813: D43.C 95.38,50.8 D10.A
N$78
  Top 0.254: U3.1 54.27,111.87 54.01,112.12 C47.1
N$80  (via drill 0.5)
  other vias: 63.01,115.88 63.01,114.88 63.01,113.88
  pour Top (no thermals): 53.51,115.38 53.51,117.88 63.51,117.88 63.51,113.38 60.51,113.38 60.51,111.88 58.51,111.88 58.51,116.88 54.51,116.88 54.51,115.38
  pour Bottom (no thermals): 57.51,116.38 57.51,113.38 63.51,113.38 63.51,116.38
N$82
  Top 0.406: C60.1 64.26,112.47 R95.1
N$84
  Top 1.016: C39.2 7.28,85.25 R92.1
N$89
  Top 1.016: C46.2 20.57,84.49 R93.1
N$90
  Top 1.016: C50.2 34.75,84.68 R94.1
N$91
  Top 0.813: D46.A 54.27,93.05 T1.1
  Bottom 0.813: T1.1 51.53,93.08
  Bottom 1.016: 51.53,93.08 44.79,93.08 42.52,90.81 42.52,77.42 C63.+ | D45.C 38.46,74.74 40.83,77.11
  Bottom 1.27: C63.+ 40.83,77.11
N$92
  Top 0.254: U3.8 62.16,110.88 C61.1
  Top 0.406: C61.1 62.26,112.47 R95.2
N$93
  Top 0.254: R96.1 R97.2
N$94
  Top 1.016: D21.C 34.91,103.37 34.9,103.36 34.95,103.31 | R94.2 34.95,103.31 | D22.A 38.99,103.34 38.96,103.36 38.92,103.31 34.95,103.31
N$95
  Top 0.254: U3.7 60.27,110.37 60.76,109.88 60.76,108.28 R98.2 R97.1
N$96  (via drill 0.5)
  Top 1.27: D46.C 45.16,93.05 44.32,92.21 44.32,91.12 v45.26,90.18
  Bottom 1.27: D47.C v45.27,90.19 v45.26,90.18
N$97
  Top 0.61: R104.2 44.16,85.08 U4.4
N$98
  Top 0.61: U4.8 52.59,88.89 T1.2
  Bottom 0.813: D47.A 53.9,90.19 T1.2
N$99  (via drill 0.5)
  Top 0.406: U4.6 v49.53,86.35 v49.53,86.34
  Top 0.61: v49.53,86.34 48.38,86.34 48,85.96 48,82.97 50.42,80.55 53.81,80.55 56.09,82.83 C65.+
  Bottom 0.406: 47.95,86.34 C64.1 | D48.C 57.44,83.93 C65.+
  Bottom 0.61: v49.53,86.34 49.53,86.44 49.25,86.72 47.96,86.72 C64.1
N$100  (via drill 0.6)
  Top 0.61: U4.5 50.37,84.63 v50.37,83.8
  Bottom 0.61: R106.1 50.31,83.86 v50.37,83.8
  Bottom 0.813: R106.1 47.95,85.16 R105.2
N$101
  Bottom 0.61: R107.1 D48.A
N$102
  Bottom 0.61: R107.2 T1.3
  Bottom 0.813: R106.2 52.01,87.38 52.68,88.05 54.24,88.05 T1.3
N$103
  pour Bottom (no thermals): 62.96,95.36 61.95,95.36 60.68,94.09 60.68,91.04 61.95,89.77 66.01,89.77 67.54,91.3 67.54,94.85 67.03,95.36
N$104
  Top 0.406: C72.1 34.91,175.36 U6.4
N$105
  Top 0.406: U6.5 33.92,176.02 34.26,176.36 36.37,176.36 36.62,176.11 C72.2
N$106
  Top 0.406: U6.1 31.38,173.41 31.06,173.08 31.06,172.28 C73.1
N$107
  Top 0.406: C73.2 29.37,173.89 30.22,174.74 U6.3
N$108
  Top 0.406: U6.12 28.54,176.02 29.92,177.4 30.2,177.68 35.23,182.71 U5.7
N$109
  Top 0.406: U5.6 38.59,183.96 35.28,183.96 27.98,176.66 U6.11
N$110
  Top 0.406: U6.2 C75.2
N$111
  Top 0.406: U6.6 33.7,176.66 C76.2
N$112
  Top 0.61: U8.8 120.04,182.6 120.04,183.73 120.88,184.56 122.01,184.56 C80.1 128.82,184.63 ISO_PULSE.1
N$113
  Top 0.61: U8.7 129.58,181.33 ISO_PULSE.2
N$114
  Top 0.61: U8.6 128.31,180.06 ISO_PULSE.3
N$115  (via drill 0.36)
  Top 0.61: C80.2 124.54,182.93 v124.56,182.91 | U8.5 122.56,178.79 v122.58,178.77 123.92,178.77 126.85,175.85 129.83,175.85 ISO_PULSE.4
  Bottom 0.61: v124.56,182.91 124.56,179.41 123.92,178.77 v122.58,178.77
NEUTRAL  (via drill 0.5, 0.6)
  Top 0.254: 49.63,17.51 49.63,18.02 49.63,18.27 50.14,18.78 50.14,19.03 50.14,19.8 | 51.53,21.98 51.53,21.45 51.66,21.32 51.16,20.81 | U3.9 58.02,111.38 58.01,111.38
  Top 1.016: 26.52,33.02 R1.1 | R3.1 78.25,44.66 L6.1 | T1.4 57.66,85.61 58.77,86.72 | 44.42,107.11 C102.-
  Top 1.27: 58.77,86.72 58.77,96.12 56.49,98.41 45.57,98.41 44.42,99.55 44.42,107.11
  Top 1.422: 26.52,33.02 26.52,22.34 31.09,17.51 47.6,17.51 | 47.6,17.51 49.63,17.51 73,17.51 77.06,21.57 77.06,23.65 NEUTRAL.TP 78.25,25.05 R3.1 | 47.6,17.51 47.6,18.02 51.53,21.98 51.83,22.5 R2.1 | 51.92,22.08 56.74,18.02 49.63,18.02 47.85,18.02 | 50.14,19.8 53.95,19.8 | 48.87,19.03 50.14,19.03 54.71,19.03 | 51.16,20.81 52.68,20.81
  Bottom 0.61: C64.2 46.19,85.16 R105.1 arc90 46.2,85.11 v46.2,83.42
  Bottom 1.016: R3.1 78.01,33.6 78.01,45.38 68.51,54.88 46.01,54.88 44.68,56.21 44.68,73.89 C63.- | D17.A 2.75,113.63 7.01,109.38 17.26,109.38 | 19.01,109.38 17.26,109.38 | 20.26,109.38 19.01,109.38 | 33.51,109.38 20.26,109.38 | 35.01,109.38 33.51,109.38 | 36.26,109.38 35.01,109.38 | D19.A 18.79,109.59 19.01,109.38 | D19.A 18.79,110.91 17.26,109.38 | D19.A 18.79,110.84 20.26,109.38 | D21.A 34.91,110.78 33.51,109.38 | D21.A 34.91,110.72 36.26,109.38 | D21.A 34.91,109.47 35.01,109.38 | 36.26,109.38 39.26,109.38 41.52,107.12 C102.-
  other vias: 56.51,111.88 57.51,111.88 56.51,110.88 56.51,109.88 57.51,110.88 57.51,109.88 64.26,107.88 62.26,107.88 63.26,107.88 71.76,96.88 71.76,97.88 70.76,97.88 70.76,96.88 73.51,102.88 73.51,101.88 72.51,102.88 47.51,106.88 48.51,106.88 49.51,106.88 62.26,101.12 64.26,101.12 63.26,101.12
  pour Top (no thermals): 43.76,108.38 46.01,108.38 47.01,109.38 50.01,109.38 50.01,106.88 56.01,106.88 56.01,112.38 55.01,113.38 55.01,116.38 58.01,116.38 58.01,108.88 59.26,108.88 59.26,107.38 58.01,107.38 58.01,103.88 58.51,103.38 74.01,103.38 74.01,96.38 66.01,96.38 62.01,100.38 49.01,100.38 43.01,106.38 43.01,107.62
  pour Bottom (no thermals): 43.76,108.38 46.01,108.38 47.01,109.38 52.51,109.38 55.51,112.38 58.01,112.38 58.01,111.38 65.01,111.38 65.01,107.38 57.51,107.38 57.51,103.38 74.01,103.38 74.01,96.38 66.01,96.38 62.01,100.38 49.01,100.38 43.01,106.38 43.01,107.62
  pour Top (no thermals): 61.51,111.38 61.51,107.38 65.01,107.38 65.01,111.38
  pour Top (no thermals): 46.58,86.22 46.58,88.76 45.95,89.39 45.06,89.39 43.53,87.87 43.53,81.39 44.93,79.99 44.93,75.67 46.58,74.02 51.92,74.02 53.19,75.29 53.19,77.71 53.44,77.96 54.58,77.96 56.11,76.44 57.12,76.44 57.63,76.94 57.63,82.03 60.3,84.69 60.3,85.45 59.54,86.22 55.34,86.22 54.96,86.6 53.57,86.6 53.19,86.22 53.19,84.69 53.69,84.18 56.11,84.18 57.38,85.45 58.27,84.56 58.27,83.3 53.69,78.72 48.74,78.72 46.71,80.75 46.71,86.09
P1+1
  Top 0.61: R5.2 16.32,43.71 16.36,43.67 16.36,41.38
  Top 1.016: 16.36,41.38 16.36,41.23 L1.2 16.24,41.27 16.36,41.38 | C39.1 3.18,65.29 2.13,64.25 2.13,43.92 4.67,41.38 16.36,41.38
P2+1  (via drill 1.1)
  Top 1.016: R8.2 41.25,44.43 41.57,44.12 L3.2 41.57,41.64 v34.65,41.64
  Bottom 1.016: C46.1 20.57,50.89 29.06,41.64 v34.65,41.64
P3+1  (via drill 1.1)
  Top 1.016: R11.2 68.13,43.71 68.17,43.67 68.11,43.61 L5.2 61.9,41.56 v61.82,41.64
  Bottom 1.016: C50.1 34.75,54.64 47.51,41.88 61.59,41.88 v61.82,41.64
  Bottom 1.27: D45.A 37.05,67.06 C50.1
PORT_DTR  (via drill 0.36)
  Top 0.406: v24.84,165.82 25.97,165.82 D51.2
  Bottom 0.406: RS1.4 21.43,173.62 22.25,172.81 22.25,167.88 24.31,165.82 v24.84,165.82
PORT_RTS
  Top 0.406: RS1.7 16.59,168.76 18.49,166.86 22.2,166.86 25.12,163.94 D50.2
PORT_RX
  Top 0.406: RS1.2 22.3,168.13 23.21,169.04 23.21,173.49 24.46,174.74 24.48,174.71 26.91,174.71 U6.14
PORT_TX
  Top 0.406: RS1.3 19.46,170.85 21.36,170.85 22.15,171.64 22.15,174.38 23.15,175.39 23.18,175.36 U6.13
R13  (via drill 0.2, 0.5)
  Top 0.254: MSP430F67791A.32 125.26,108.88 126.76,110.38 127.25,110.88 v128,110.88 v128.01,110.88 | R46.2 v132.26,116.38 R43.1
  Bottom 0.254: v132.26,116.38 132.26,114.36 128.88,110.98 128.11,110.98 v128.01,110.88
R23  (via drill 0.2, 0.5)
  Top 0.254: MSP430F67791A.31 125.51,108.38 126.51,109.38 v128.01,109.38 | R43.2 v132.26,112.38 R42.1
  Bottom 0.254: v132.26,112.38 132.26,112.33 129.39,109.46 128.09,109.46 v128.01,109.38
R33  (via drill 0.2, 0.5)
  Top 0.254: MSP430F67791A.30 126.51,107.88 v127.01,108.38 | v132.26,108.38 R42.2 133.16,109.53 133.88,110.25 C49.1
  Bottom 0.254: v127.01,108.38 v132.26,108.38
REACT
  Top 0.254: LED_REACT.K 85.55,170.38 102.51,170.38 110.51,162.38 110.51,150.88 120.51,140.88 MSP430F67791A.42
  Top 0.61: JP11.1 92.99,175.9 97.86,180.78 97.89,180.78 98.63,181.52 108.61,181.52 110.03,180.09 114.28,180.09 U8.3
  Bottom 0.254: JP11.1 83.79,168.83 LED_REACT.K
RESET  (via drill 0.2)
  Top 0.254: C53.2 33.66,132.81 | RESET.1 38.15,131.05 36.91,132.29 33.79,132.29 C53.2 | C53.2 32.32,132.41 31.68,131.76 31.68,131.06 31.67,131.06
  Top 0.305: C53.2 R51.2 | v31.67,126.06 31.67,131.06
  Bottom 0.254: v31.67,126.06 30.67,125.06 26.17,125.06 25.42,125.81 25.42,128.06 24.4,129.08 JP5.3 22.9,129.08 19.18,132.8 | JTAG.11 14.66,131.63 15.83,132.8 19.18,132.8 | 19.18,132.8 19.18,132.81
RS232_RXD  (via drill 0.2, 0.5)
  Top 0.254: MSP430F67791A.16 122.01,100.88 112.63,110.25 v110.63,110.25
  Top 0.406: RX_EN.2 56.9,176.62 54.13,173.85 51.23,173.85 48.61,171.23 48.61,160 52.02,156.6 54.48,156.6 v54.51,156.62
  Bottom 0.254: v54.51,156.62 60.26,150.88 87.51,150.88 104.76,133.62 108.76,133.62 109.51,132.88 109.51,111.38 v110.63,110.25
RS232_TXD  (via drill 0.2, 0.5)
  Top 0.254: MSP430F67791A.17 122.51,101.38 113.01,110.88 111.01,110.88 v110.51,111.38
  Top 0.406: TX_EN.2 57.73,184.82 60.98,181.57 60.98,175.4 58.11,172.53 52.7,172.53 50.21,170.04 50.21,160.97 52.06,159.12 v53.76,159.12
  Bottom 0.254: v110.51,111.38 110.51,133.38 109.26,134.62 105.26,134.62 88.01,151.88 61.01,151.88 v53.76,159.12
RTCCLK  (via drill 0.36)
  Top 0.254: MSP430F67791A.92 110.52,98.38 v110.54,98.36
  Bottom 0.254: v110.54,98.36 110.56,98.36 122.38,110.17 122.38,153.04 114.86,160.56 114.86,174.3 106.63,182.53 106.04,183.12 104.8,184.36 RTC.2
S0
  Top 0.254: MSP430F67791A.87 101.01,100.88 94.01,107.88 94.01,120.38 91.01,123.38 62.74,123.38 53.58,132.53 LCD1.1
S1
  Top 0.254: MSP430F67791A.86 101.26,101.38 94.51,108.12 94.51,120.62 91.26,123.88 64.76,123.88 56.1,132.53 LCD1.2
S2
  Top 0.254: MSP430F67791A.85 101.51,101.88 95.01,108.38 95.01,120.88 91.51,124.38 66.76,124.38 58.6,132.53 LCD1.3
S3
  Top 0.254: MSP430F67791A.84 101.76,102.38 95.51,108.62 95.51,121.12 91.76,124.88 68.76,124.88 LCD1.4
S4
  Top 0.254: MSP430F67791A.83 102.01,102.88 96.01,108.88 96.01,121.38 92.01,125.38 70.76,125.38 63.64,132.49 LCD1.5
S5
  Top 0.254: MSP430F67791A.82 102.26,103.38 96.51,109.12 96.51,121.62 92.26,125.88 72.76,125.88 66.18,132.45 LCD1.6
S6
  Top 0.254: MSP430F67791A.81 102.51,103.88 97.01,109.38 97.01,121.88 92.51,126.38 74.76,126.38 68.72,132.41 LCD1.7
S7
  Top 0.254: MSP430F67791A.80 102.76,104.38 97.51,109.62 97.51,122.12 92.76,126.88 76.76,126.88 71.26,132.37 LCD1.8
S8
  Top 0.254: MSP430F67791A.79 103.01,104.88 98.01,109.88 98.01,122.38 93.01,127.38 78.76,127.38 73.8,132.33 LCD1.9
S9
  Top 0.254: MSP430F67791A.78 103.26,105.38 98.51,110.12 98.51,122.62 93.26,127.88 80.76,127.88 76.34,132.29 LCD1.10
S10
  Top 0.254: MSP430F67791A.77 103.51,105.88 99.01,110.38 99.01,122.88 93.51,128.38 82.76,128.38 78.88,132.25 LCD1.11
S11
  Top 0.254: MSP430F67791A.76 103.76,106.38 99.51,110.62 99.51,123.12 93.76,128.88 84.76,128.88 81.42,132.21 LCD1.12
S12
  Top 0.254: MSP430F67791A.75 104.01,106.88 100.01,110.88 100.01,123.38 94.01,129.38 86.76,129.38 83.96,132.2 LCD1.13
S13
  Top 0.254: MSP430F67791A.74 104.26,107.38 100.51,111.12 100.51,123.62 94.26,129.88 88.76,129.88 86.5,132.13 LCD1.14
S14
  Top 0.254: MSP430F67791A.73 104.51,107.88 101.01,111.38 101.01,123.88 94.51,130.38 90.76,130.38 89.04,132.12 LCD1.15
S15
  Top 0.254: MSP430F67791A.72 104.76,108.38 101.51,111.62 101.51,124.12 94.76,130.88 92.76,130.88 91.58,132.08 LCD1.16
S16
  Top 0.254: MSP430F67791A.71 105.01,108.88 102.01,111.88 102.01,124.38 94.12,132.29 LCD1.17
S17
  Top 0.254: MSP430F67791A.68 104.26,110.38 102.51,112.12 102.51,124.62 96.66,130.43 LCD1.18
S18
  Top 0.254: MSP430F67791A.67 104.51,110.88 103.01,112.38 103.01,124.88 99.2,128.71 LCD1.19
S19
  Top 0.254: MSP430F67791A.66 104.76,111.38 103.51,112.62 103.51,125.12 101.74,126.92 LCD1.20
S20
  Top 0.254: MSP430F67791A.65 105.01,111.88 104.01,112.88 104.01,132.26 LCD1.21
S21
  Top 0.254: MSP430F67791A.64 109.51,131.88 109.01,132.38 108.81,132.57 106.86,132.57 LCD1.22
S22  (via drill 0.36)
  Top 0.254: MSP430F67791A.63 110.01,132.38 107.01,135.38 v106.51,135.38
  Bottom 0.254: v106.51,135.38 106.51,162.19 LCD1.23
S23  (via drill 0.36)
  Top 0.254: MSP430F67791A.62 110.51,132.62 106.76,136.38 v105.51,136.38
  Bottom 0.254: v105.51,136.38 105.51,161.28 LCD1.24
S24  (via drill 0.36)
  Top 0.254: MSP430F67791A.61 111.01,132.88 106.51,137.38 v104.51,137.38
  Bottom 0.254: v104.51,137.38 104.51,149.38 91.58,162.26 LCD1.29
S25  (via drill 0.36)
  Top 0.254: MSP430F67791A.60 111.51,133.12 106.26,138.38 v103.51,138.38
  Bottom 0.254: v103.51,138.38 103.51,149.62 93.26,159.88 91.51,159.88 89.04,162.34 LCD1.30
S26  (via drill 0.36)
  Top 0.254: MSP430F67791A.59 112.01,133.38 106.01,139.38 v102.51,139.38
  Bottom 0.254: v102.51,139.38 102.51,149.88 93.01,159.38 89.51,159.38 86.5,162.38 LCD1.31
S27  (via drill 0.36)
  Top 0.254: MSP430F67791A.58 112.51,133.62 105.76,140.38 v101.51,140.38
  Bottom 0.254: v101.51,140.38 101.51,150.12 92.76,158.88 87.51,158.88 83.96,162.42 LCD1.32
S28  (via drill 0.36)
  Top 0.254: MSP430F67791A.57 113.01,133.88 105.51,141.38 v100.51,141.38
  Bottom 0.254: v100.51,141.38 100.51,150.38 92.51,158.38 85.51,158.38 81.42,162.46 LCD1.33
S29  (via drill 0.36)
  Top 0.254: MSP430F67791A.56 113.51,134.12 105.26,142.38 v99.51,142.38
  Bottom 0.254: v99.51,142.38 99.51,150.62 92.26,157.88 83.51,157.88 LCD1.34
S30  (via drill 0.36)
  Top 0.254: MSP430F67791A.55 114.01,134.38 105.01,143.38 v98.51,143.38
  Bottom 0.254: v98.51,143.38 98.51,150.88 92.01,157.38 81.51,157.38 76.38,162.5 LCD1.35
S31  (via drill 0.36)
  Top 0.254: MSP430F67791A.54 114.51,134.62 104.76,144.38 v97.51,144.38
  Bottom 0.254: v97.51,144.38 97.51,151.12 91.76,156.88 79.51,156.88 73.88,162.5 LCD1.36
S32  (via drill 0.36)
  Top 0.254: MSP430F67791A.53 115.01,134.88 104.51,145.38 v96.51,145.38
  Bottom 0.254: v96.51,145.38 96.51,151.38 91.51,156.38 77.51,156.38 71.38,162.5 LCD1.37
S33  (via drill 0.36)
  Top 0.254: MSP430F67791A.52 115.51,135.12 104.26,146.38 v95.51,146.38
  Bottom 0.254: v95.51,146.38 95.51,151.62 91.26,155.88 75.51,155.88 68.88,162.5 LCD1.38
S34  (via drill 0.36)
  Top 0.254: MSP430F67791A.51 116.01,135.38 104.01,147.38 v94.51,147.38
  Bottom 0.254: v94.51,147.38 94.51,151.88 91.01,155.38 73.26,155.38 66.18,162.45 LCD1.39
S35  (via drill 0.36)
  Top 0.254: MSP430F67791A.50 116.51,135.62 103.76,148.38 v93.51,148.38
  Bottom 0.254: v93.51,148.38 93.51,152.12 90.76,154.88 71.26,154.88 LCD1.40
S36  (via drill 0.36)
  Top 0.254: MSP430F67791A.49 117.01,135.88 103.51,149.38 v92.51,149.38
  Bottom 0.254: v92.51,149.38 92.51,152.38 90.51,154.38 69.26,154.38 61.13,162.5 LCD1.41
S37  (via drill 0.36)
  Top 0.254: MSP430F67791A.48 117.51,136.12 103.26,150.38 v91.51,150.38
  Bottom 0.254: v91.51,150.38 91.51,152.62 90.26,153.88 67.26,153.88 58.63,162.5 LCD1.42
S38  (via drill 0.36)
  Top 0.254: MSP430F67791A.47 118.01,136.38 103.01,151.38 v90.51,151.38
  Bottom 0.254: v90.51,151.38 90.51,152.88 90.01,153.38 65.26,153.38 56.13,162.5 LCD1.43
S39  (via drill 0.36)
  Top 0.254: MSP430F67791A.46 118.51,136.62 102.76,152.38 v89.51,152.38
  Bottom 0.254: v89.51,152.38 89.01,152.88 63.01,152.88 53.48,162.4 LCD1.44
TCK
  Top 0.254: R48.1 21.62,131.09 22.14,131.62 JP6.3
  Bottom 0.254: JP6.3 22.91,131.62 19.1,135.43 15.92,135.43 JTAG.7
TDI
  Bottom 0.254: JP8.3 22.91,136.7 19.05,140.56 15.88,140.56 JTAG.3
TDO
  Top 0.254: JP9.3 25.45,137.97 27.36,137.97 27.99,137.33 27.99,130.35 JP5.1
  Bottom 0.254: JP9.3 22.91,139.24 19.1,143.05 15.93,143.05 JTAG.1
TEST/SBWTCK  (via drill 0.36)
  Top 0.254: JTAG.8 19.1,134.79 19.1,126.54 20.37,125.27 22.91,125.27 JP4.3 JP4.2 26.72,126.51 27.82,125.41 28.17,125.06 28.2,125.03 33.27,125.03 36.12,127.88 55.54,127.88 60.58,122.83 90.76,122.88 93.51,120.12 93.51,107.12 94.55,106.08 v94.74,106.08 | MSP430F67791A.97 101.51,95.88 v100.88,95.25
  Bottom 0.254: v100.88,95.25 100.81,95.18 99.06,95.18 95.25,98.99 95.25,105.57 v94.74,106.08
TMS
  Bottom 0.254: JP7.3 22.91,134.16 19.14,137.93 15.96,137.93 JTAG.5
UART_RX
  Top 0.406: U5.2 49.98,182.71 50.44,182.25 54.33,182.25 RX_EN.1
UART_TX
  Top 0.406: U5.3 53.52,183.98 TX_EN.1
V1+
  Top 0.254: MSP430F67791A.103 109.51,90.88 102.51,83.88
  Top 0.406: 102.51,83.88 102.51,74.88 100.51,72.88 54.76,72.88 47.26,65.38 47.26,62.88 47.96,62.17 C8.1
  Top 0.679: C8.1 C1.1 49.11,59.48 R14.1
V1-
  Top 0.254: MSP430F67791A.104 110.01,90.62 103.51,84.12 103.51,83.88
  Top 0.406: 103.51,83.88 103.51,74.38 101.01,71.88 61.51,71.88 55.01,65.38 R32.1
  Top 0.61: 54.66,64.08 R32.1
  Top 0.679: C8.2 C9.1 54.66,64.08
V2+
  Top 0.254: MSP430F67791A.105 110.51,90.38 104.51,84.38 104.51,83.88
  Top 0.406: 104.51,83.88 104.51,73.88 101.51,70.88 64.76,70.88 59.26,65.38 59.26,62.88 59.96,62.17 C10.1
  Top 0.61: C2.1 C10.1
  Top 0.679: R16.1 61.11,59.48 C2.1
V2-
  Top 0.254: MSP430F67791A.106 111.01,90.12 105.51,84.62 105.51,83.88
  Top 0.406: 105.51,83.88 105.51,73.38 102.01,69.88 71.51,69.88 66.91,65.28 66.91,64.08
  Top 0.61: 66.91,64.08 R33.1
  Top 0.679: C10.2 C11.1 66.91,64.08
V3+
  Top 0.254: MSP430F67791A.107 111.51,89.88 106.51,84.88 106.51,83.88
  Top 0.406: 106.51,83.88 106.51,72.88 102.51,68.88 75.01,68.88 71.51,65.38 71.51,62.88 72.21,62.17 C12.1
  Top 0.679: C12.1 C3.1 73.36,59.48 R18.1
V3-
  Top 0.254: MSP430F67791A.108 112.01,89.62 107.51,85.12 107.51,83.88
  Top 0.406: 107.51,83.88 107.51,72.38 103.01,67.88 83.92,67.88 83.92,67.8 83.67,67.55 83.67,65.77 81.87,63.98 R34.1
  Top 0.61: 78.66,64.08 R34.1
  Top 0.679: C12.2 C13.1 78.66,64.08
VASYS1/2
  Top 0.254: C23.1 112.01,85.12 111.86,84.97 C22.1 110.51,85.88 113.51,88.88 MSP430F67791A.111 113.51,93.38 114.01,93.88 118.51,93.88 119.01,93.38 MSP430F67791A.122 119.01,89.48 120.61,87.88 122.51,87.88 122.75,87.64 C32.1
  Top 0.406: C32.1 122.75,86.64 122.76,86.62 C28.1
VCC_ISO
  Bottom 0.813: C67.1 C66.+
  Bottom 1.016: C67.1 82.78,93.56 C68.1 83.32,93.02 R108.2
  pour Bottom (no thermals): 82.78,92.31 85.82,92.31 86.08,92.57 86.08,93.58 84.81,94.85 84.81,104 83.54,105.27 81.76,105.27 81.51,105.01 81.51,97.39 80.24,96.12 74.9,96.12 73.38,94.6 69.82,94.6 69.31,94.09 69.31,92.82 70.08,92.06 78.2,92.06 78.46,92.31
VCC_PL  (via drill 0.6)
  Top 1.016: JP3.3 77.55,103.84
  other vias: 66.01,104.62 67.26,104.62 67.19,106.14 65.94,106.14
  pour Top (no thermals): 60.01,105.38 61.51,105.38 61.51,106.62 78.51,106.62 78.51,102.88 77.01,102.88 75.76,104.12 60.01,104.12
  pour Bottom (no thermals): 58.01,106.62 58.01,104.12 75.76,104.12 77.01,102.88 78.51,102.88 78.51,106.62
VCC_RS232
  Top 0.406: U6.16 27.07,173.26 C74.1 27.07,169.68 27.66,169.1 34,169.1 C71.1 | C71.1 34.04,167.82 U7.5 34.03,167.78 35.25,167.78 35.58,167.44 JP14.1 | U5.8 37.11,181.44 36.68,181.01 36.68,180.21 C77.1 38.08,180.16 38.63,179.61 38.63,172.12 36.95,170.44 34.54,170.44 34.06,169.96 34.06,169.07 C71.1
VCORE
  Top 0.254: C38.1 123.51,91.38 123.51,91.58 MSP430F67791A.128
VREF
  Top 0.254: MSP430F67791A.113 114.51,89.62 114.01,89.12 114.01,88.38 113.51,87.88 C30.1
VSUPPLY
  Top 0.254: U3.2 51.26,111.38 R35.2
  Bottom 1.016: D18.C 7.25,116.11 10.01,118.88 21.76,118.88 | 21.76,118.88 23.01,118.88 | 23.01,118.88 24.51,118.88 | 24.51,118.88 37.76,118.88 | 37.76,118.88 39.51,118.88 | 39.51,118.88 40.76,118.88 | 40.76,118.88 41.51,118.88 44.43,115.95 C102.+ | D22.C 39.28,118.65 39.51,118.88 | D22.C 39.28,117.4 40.76,118.88 | D22.C 39.28,117.35 37.76,118.88 | D20.C 23.07,118.81 23.01,118.88 | D20.C 23.07,117.44 24.51,118.88 | D20.C 23.07,117.56 21.76,118.88
  pour Top (no thermals): 43.51,113.38 45.01,113.38 46.01,112.38 51.51,112.38 51.51,110.88 50.01,110.88 50.01,110.38 44.51,110.38 43.01,111.88 43.01,112.88
XIN
  Top 0.254: MSP430F67791A.1 126.01,93.38 126.86,92.53 128.41,92.53 XT1.P2 130.51,92.38 131.41,91.47 C37.1 131.41,90.97
XOUT
  Top 0.254: XT1.P1 128.41,95.06 | MSP430F67791A.2 126.01,93.88 127.01,94.88 XT1.P1 | XT1.P1 130.55,94.88 131.37,95.69 131.37,96.34 C40.1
